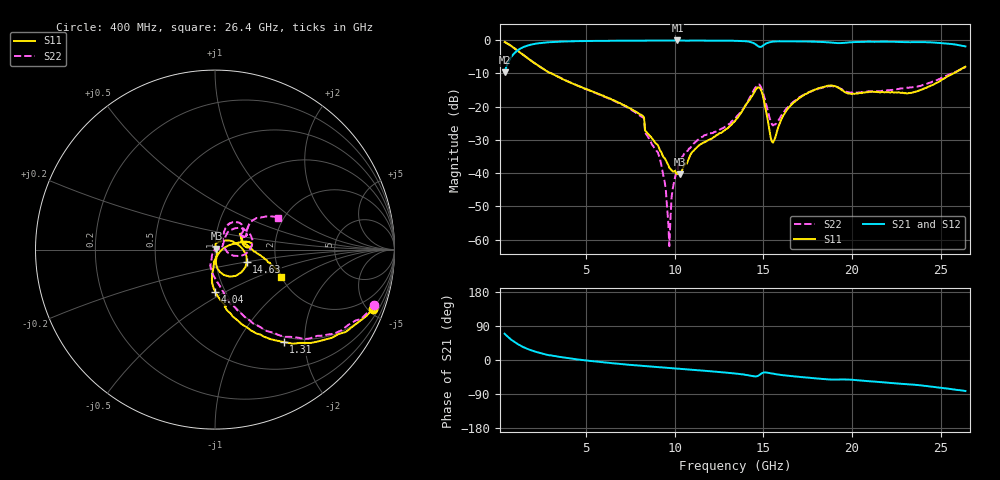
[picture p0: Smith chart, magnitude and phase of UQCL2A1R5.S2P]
! AVX Corporation
! Date:  10/27/06
! Part No:  UQCL2A1R5
! Description:  Ultra Low ESR Microwave capacitors
! Mounting Orientation:  Horizontal
# GHZ S DB R 50
! Freq  |S11|  S11 Ph  |S21|  S21 Ph  |S12|  S12 Ph  |S22|  S22 Ph
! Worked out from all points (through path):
!   401 points, 400 MHz to 26.4 GHz, reference 50 ohm
!   highest |S21| = -0.07 dB at 10.15 GHz (marker M1); lowest = -9.6 dB at 400 MHz (marker M2)
!   group delay of S21, straight-line fit = 11.2 ps
!   lowest |S11| = -40.4 dB at 10.28 GHz (marker M3), VSWR 1.02, Z = 50.8 + j0.569 ohm
!   |S11| at or under -10 dB: 3.045 GHz to 25.71 GHz (22.66 GHz wide, 158 % of centre)
!   |S22| runs from -62.0 to -0.5 dB; largest |S21 - S12| = 0.0069
!   S11 on the Smith chart (normalised r, x): 400 MHz: 0.96, -5.34; 1.31 GHz: 0.91, -1.59; 4.04 GHz: 0.90, -0.45; 14.63 GHz: 1.41, -0.20; 26.4 GHz: 2.00, -0.72
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0.4  -0.55 -20.6  -9.64 69.3  -9.65 69.3  -0.53 -19.3
1.31  -3.85 -53.4  -2.47 37.6  -2.48 37.8  -3.85 -49.2
2.35  -7.81 -73.0  -0.88 19.0  -0.88 19.1  -7.84 -66.5
4.04  -12.59 -89.7  -0.34 4.5  -0.35 4.3  -12.56 -79.3
4.755  -14.16 -93.6  -0.27 0.1  -0.27 0.1  -14.22 -84.0
8.135  -22.53 -94.7  -0.12 -15.5  -0.13 -15.5  -23.04 -107.2
8.46  -27.98 -77.6  -0.13 -16.5  -0.14 -16.6  -28.83 -119.8
9.11  -32.39 -62.6  -0.13 -19.1  -0.14 -19.1  -34.76 -126.8
9.37  -35.22 -50.0  -0.13 -19.9  -0.14 -20.0  -41.12 -131.4
9.695  -38.39 -27.0  -0.11 -21.1  -0.12 -21.1  -61.97 -26.7
10.15  -40.24 19.0  -0.07 -22.9  -0.09 -23.0  -38.84 20.3
10.28  -40.40 35.9  -0.08 -23.5  -0.09 -23.5  -36.88 19.4
11.255  -32.20 83.3  -0.10 -26.9  -0.11 -26.9  -30.19 12.2
13.4  -24.32 50.1  -0.19 -35.8  -0.21 -35.8  -23.56 42.5
14.635  -14.47 -20.7  -1.51 -43.0  -1.50 -43.1  -13.61 29.0
14.96  -16.46 -70.6  -1.71 -33.8  -1.70 -33.9  -15.47 -9.2
15.545  -30.80 -34.2  -0.43 -36.2  -0.43 -36.2  -25.65 14.8
16.39  -20.54 17.3  -0.32 -41.5  -0.32 -41.5  -20.09 61.6
17.755  -15.18 14.8  -0.42 -47.6  -0.43 -47.6  -15.29 59.2
22.11  -15.66 30.3  -0.46 -60.3  -0.45 -60.3  -15.00 23.8
23.67  -15.39 11.9  -0.57 -65.9  -0.57 -65.9  -14.00 28.4
26.4  -7.97 -22.1  -1.86 -81.9  -1.87 -82.2  -8.12 26.6
